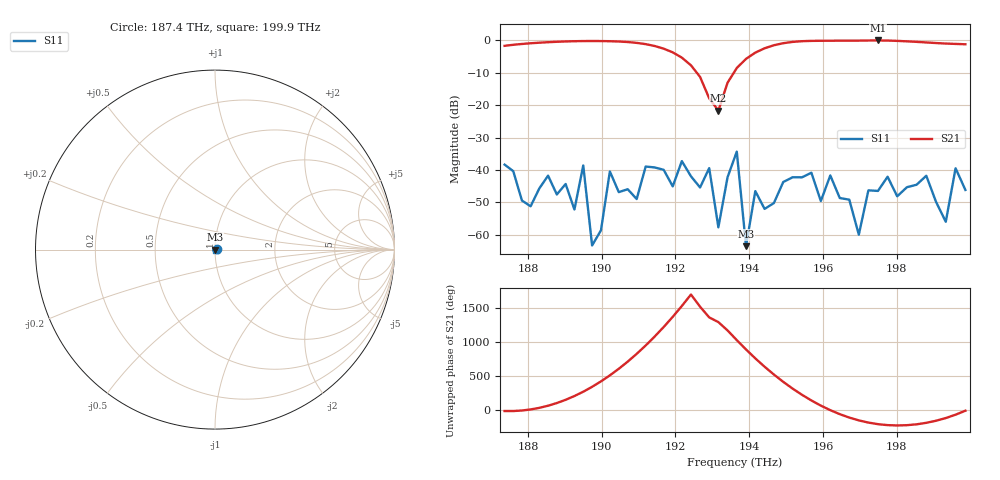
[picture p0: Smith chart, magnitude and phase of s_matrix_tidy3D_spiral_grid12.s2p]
[Version] 2.0
# Hz S RI
[Number of Ports] 2
[Two-Port Data Order] 12_21
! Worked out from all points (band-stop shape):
!   51 points, 187.4 THz to 199.9 THz, reference 50 ohm
!   highest |S21| = -0.05 dB at 197.5 THz (marker M1); lowest = -21.7 dB at 193.2 THz (marker M2)
!   |S21| within 3 dB of the highest: start of sweep to 191.8 THz; 194.3 THz to end of sweep
!   lowest |S11| = -63.5 dB at 193.9 THz (marker M3), VSWR 1.00, Z = 49.9 + j0.0445 ohm
!   |S11| at or under -10 dB: start of sweep to end of sweep
!   S12 and S22 are empty: the file has one direction only
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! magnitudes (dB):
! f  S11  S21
! 187.4 THz  -38.3  -1.7
! 189.3 THz  -52.2  -0.3
! 189.5 THz  -38.6  -0.2
! 189.7 THz  -63.3  -0.2
! 190.2 THz  -40.4  -0.3
! 191 THz  -48.9  -0.8
! 191.7 THz  -39.9  -2.6
! 192.9 THz  -39.4  -17.9
! 193.2 THz  -57.7  -21.7
! 193.7 THz  -34.3  -8.5
! 193.9 THz  -63.5  -5.7
! 194.2 THz  -46.5  -3.8
! 195.7 THz  -40.8  -0.2
! 195.9 THz  -49.6  -0.1
! 196.2 THz  -41.7  -0.1
! 197 THz  -59.9  -0.1
! 197.5 THz  -46.4  0.0
! 198 THz  -48.1  -0.2
! 198.8 THz  -41.8  -0.7
! 199.3 THz  -55.9  -1.0
! 199.6 THz  -39.5  -1.1
! 199.9 THz  -46.1  -1.2
